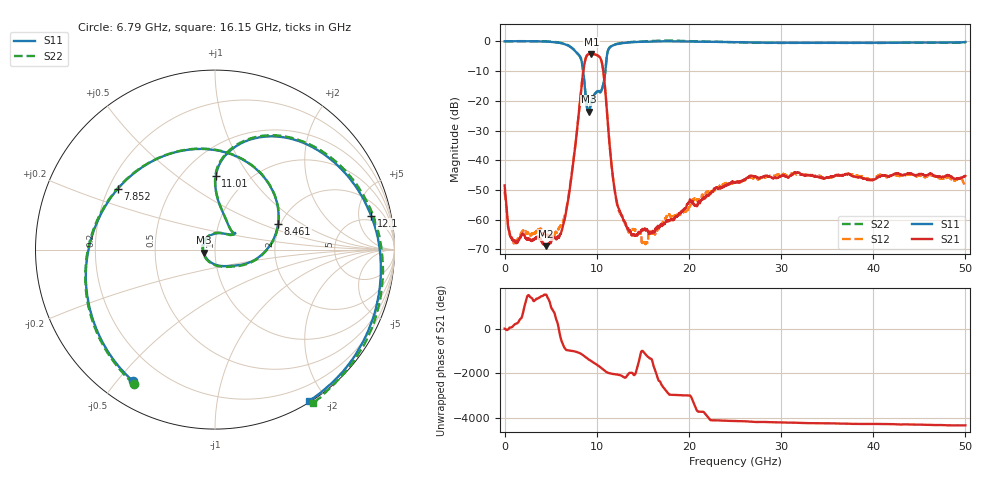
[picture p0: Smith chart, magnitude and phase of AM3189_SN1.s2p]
!Agilent Technologies,E8364B,MY43040894,A.07.50.67
!Agilent E8364B: A.07.50.67
!Date: Friday, July 10, 2020 10:53:11
!Correction: S11(Full 2 Port(1,2))
!S21(Full 2 Port(1,2))
!S12(Full 2 Port(1,2))
!S22(Full 2 Port(1,2))
!S2P File: Measurements: S11, S21, S12, S22:
# Hz S  dB  R 50
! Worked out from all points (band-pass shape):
!   3201 points, 10 MHz to 50 GHz, reference 50 ohm
!   highest |S21| = -4.24 dB at 9.43 GHz (marker M1); lowest = -68.9 dB at 4.462 GHz (marker M2)
!   |S21| within 3 dB of the highest: 8.691 GHz to 10.57 GHz (1.876 GHz wide, 19.5 % of centre)
!   lowest |S11| = -23.7 dB at 9.118 GHz (marker M3), VSWR 1.14, Z = 44 - j1.52 ohm
!   |S11| at or under -10 dB: 8.529 GHz to 10.94 GHz (2.408 GHz wide, 24.7 % of centre)
!   |S22| runs from -23.2 to 0.3 dB; largest |S21 - S12| = 0.0067
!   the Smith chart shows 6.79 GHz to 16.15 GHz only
!   S11 on the Smith chart (normalised r, x): 6.79 GHz: 0.10, -0.55; 7.852 GHz: 0.24, +0.27; 8.461 GHz: 1.94, +0.65; 11.01 GHz: 0.72, +0.71; 12.1 GHz: 3.99, +7.20; 16.15 GHz: 0.01, -1.79
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1e7  -0.00 -0.9  -48.47 7.3  -50.49 178.9  0.02 -1.0
8.379594e8  0.02 -8.8  -66.81 87.2  -66.35 -55.5  0.04 -8.5
4.462234e9  -0.09 -55.8  -68.91 96.0  -64.99 55.2  0.00 -55.3
6.789894e9  -1.27 -122.1  -55.54 123.8  -54.86 129.9  -1.16 -121.1
7.852181e9  -3.89 148.2  -30.39 37.3  -30.36 37.5  -3.83 149.4
8.352081e9  -6.53 50.0  -15.06 -55.7  -15.06 -55.9  -6.48 50.6
8.461434e9  -8.40 22.3  -12.04 -85.8  -12.04 -85.9  -8.33 22.7
8.805116e9  -19.10 -56.3  -5.75 166.2  -5.75 166.1  -18.57 -55.0
9.117553e9  -23.69 -164.8  -4.32 69.2  -4.31 69.2  -23.25 -162.3
9.429991e9  -20.64 78.8  -4.24 -15.8  -4.24 -15.9  -20.42 80.7
9.711184e9  -18.06 42.6  -4.32 -89.7  -4.32 -89.7  -18.21 41.5
1.0008e10  -16.94 38.6  -4.61 -169.0  -4.62 -169.1  -17.03 37.7
1.033606e10  -17.16 42.5  -5.36 95.6  -5.36 95.5  -17.11 41.7
1.10078e10  -7.74 89.4  -19.32 -126.9  -19.29 -126.9  -7.89 89.9
1.210133e10  -1.01 12.2  -52.80 113.3  -53.07 114.4  -0.90 12.4
1.372601e10  -0.33 -25.7  -64.67 -170.3  -63.31 -38.5  -0.21 -25.5
1.61474e10  -0.05 -58.3  -64.14 160.3  -64.47 65.6  0.13 -57.4
1.667854e10  -0.03 -64.1  -62.27 -121.7  -62.71 155.3  0.20 -63.2
2.5005e10  -0.31 -135.2  -47.48 -179.7  -47.21 -179.2  -0.33 -133.7
3.334708e10  -0.51 170.2  -45.04 83.2  -45.07 82.8  -0.53 173.9
4.167354e10  -0.45 125.1  -45.49 40.1  -45.43 38.3  -0.51 128.3
5e10  -0.21 82.0  -45.30 -15.6  -49.04 -12.1  -0.50 84.8
